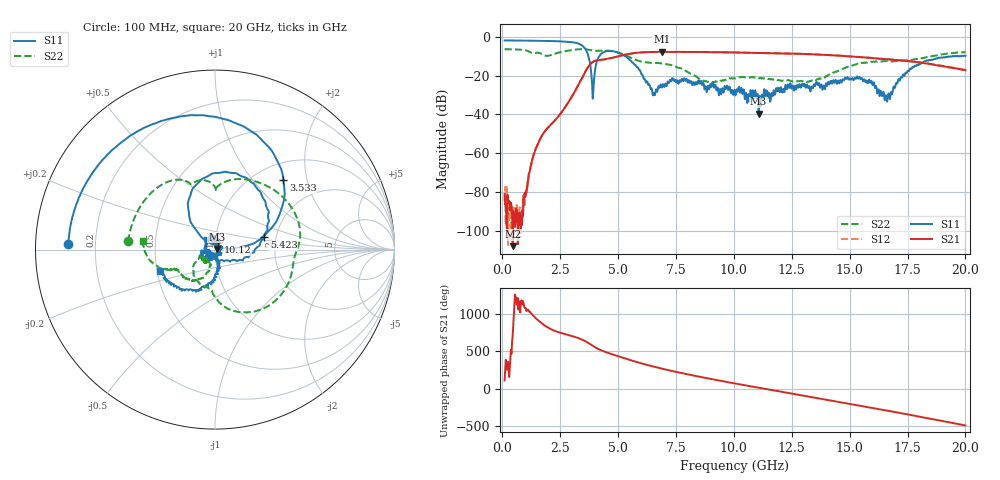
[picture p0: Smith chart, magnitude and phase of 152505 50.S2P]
!  2-Port S-parameters saved by WinCal
! VAR MeasName=S-Parameters (CALIBRATED_DATA) read from VNA (N5230C)
! VAR MeasDate=4/10/2015 9:33:35 AM
! VAR NAME=152505 50
! VAR FILENAME=152505 50.S2P
! VAR DATE=4/10/2015 9:33:35 AM
! VAR PHYS_PORTS=1,2
# Hz S DB R 50
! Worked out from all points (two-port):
!   801 points, 100 MHz to 20 GHz, reference 50 ohm
!   highest |S21| = -7.61 dB at 6.891 GHz (marker M1); lowest = -108.1 dB at 448.2 MHz (marker M2)
!   |S21| within 3 dB of the highest: 4.781 GHz to 15.73 GHz (10.94 GHz wide, 107 % of centre)
!   lowest |S11| = -39.6 dB at 11.07 GHz (marker M3), VSWR 1.02, Z = 51 + j0.363 ohm
!   |S11| at or under -10 dB: 3.721 GHz to 4.182 GHz (461.5 MHz wide, 11.7 % of centre); 5.313 GHz to 19.34 GHz (14.03 GHz wide, 114 % of centre); 19.38097 GHz to 19.4319 GHz (50.93 MHz wide, 0.262 % of centre)
!   |S22| runs from -23.7 to -6.2 dB; largest |S21 - S12| = 0.0057
!   S11 on the Smith chart (normalised r, x): 100 MHz: 0.10, +0.02; 3.533 GHz: 1.33, +1.45; 5.423 GHz: 1.73, +0.26; 10.12 GHz: 1.03, +0.09; 20 GHz: 0.52, -0.14
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1e8  -1.75 177.6  -81.12 107.6  -84.59 -96.4  -6.29 174.6
4.4825e8  -1.77 169.3  -108.07 -10.7  -96.32 67.4  -6.34 155.8
9.955e8  -1.83 156.1  -82.58 -3.3  -82.88 17.3  -6.79 123.5
1.617375e9  -1.94 140.1  -53.12 175.7  -53.21 176.3  -8.30 96.3
2.83625e9  -2.44 98.0  -34.06 -2.3  -34.05 -2.5  -7.03 57.7
3.43325e9  -4.24 56.7  -21.30 -62.9  -21.34 -62.9  -6.21 23.7
3.53275e9  -5.31 45.4  -19.03 -77.3  -19.06 -77.4  -6.22 17.3
3.905875e9  -31.81 46.5  -12.86 -147.9  -12.88 -148.0  -6.95 -3.0
4.353625e9  -7.93 99.9  -11.62 141.6  -11.66 141.1  -6.95 -23.1
5.42325e9  -10.97 14.2  -8.79 31.2  -8.80 31.4  -9.93 -81.4
6.492875e9  -29.52 -104.8  -7.69 -63.8  -7.70 -63.5  -13.36 -101.8
6.741625e9  -25.39 179.6  -7.65 -82.7  -7.64 -82.9  -13.40 -109.3
6.890875e9  -26.06 169.9  -7.61 -93.8  -7.65 -93.8  -13.64 -113.5
8.259e9  -23.26 92.9  -7.68 174.1  -7.70 174.3  -19.66 -152.0
1.005e10  -29.28 81.8  -7.94 67.6  -7.98 67.6  -21.34 -124.2
1.012462e10  -26.96 66.1  -7.97 63.4  -8.00 63.6  -21.14 -124.9
1.106988e10  -39.59 19.8  -8.22 10.7  -8.19 10.7  -21.21 -135.4
1.338325e10  -25.93 -137.5  -8.91 -116.4  -8.86 -116.2  -22.33 -117.9
1.539812e10  -21.26 -157.7  -10.26 132.3  -10.28 131.8  -13.68 -124.4
1.669162e10  -29.11 -95.0  -11.52 60.5  -11.54 60.2  -12.44 -147.6
1.7811e10  -14.80 -94.4  -12.82 -4.3  -12.78 -4.7  -11.58 -155.3
2e10  -9.68 -159.2  -17.10 -134.6  -17.07 -134.4  -7.82 173.0
